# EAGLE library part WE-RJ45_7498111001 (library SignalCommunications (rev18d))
Order Code 7498111001 Design SMD xBase-T 10/100/1000 Base-T Ports 1x1 Application Standard Tab Position UP LED (Left-Right) NONE EMI Fingers Yes Details see: http://katalog.we-online.de/en/pbs/WE-LAN_RJ45/7498111001? Updated by Yingchun Shan 2016-08-23 2014 (C) Würth Elektronik
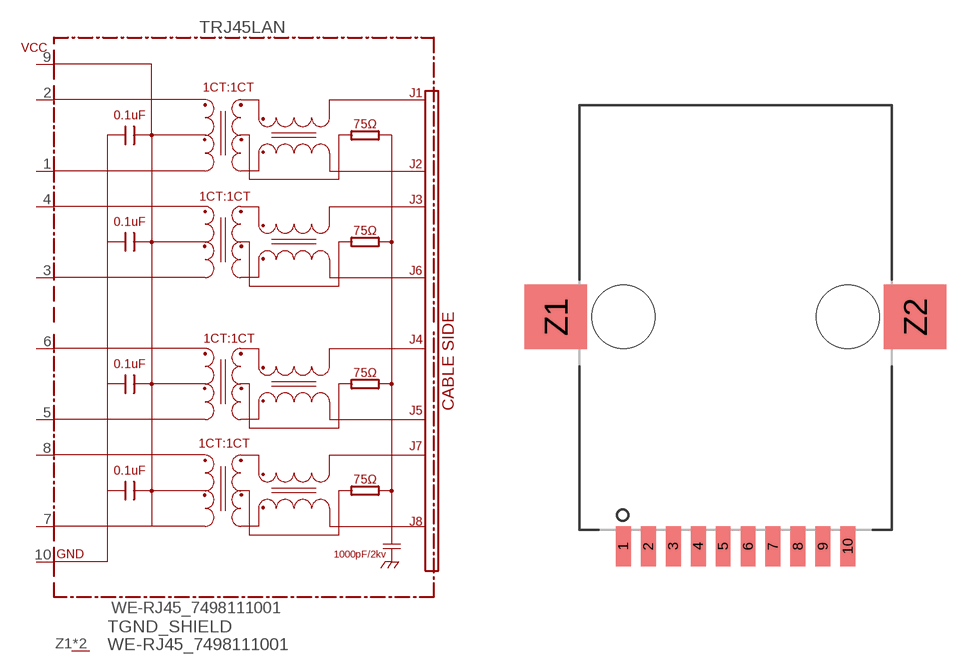
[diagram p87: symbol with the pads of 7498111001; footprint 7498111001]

Designator prefix T; gates RJ45LAN=7498111001 GND_SHIELD=GNDPIN

## WE-RJ45_7498111001 (COMPANY-URL: http://www.we-online.de; CREATED-BY: Christin Zierenner; CREATED-DATE: AUG 2012; DATASHEET-URL: http://katalog.we-online.de/kataloge/eisos/media/pdf/7498111001.pdf; MANUFACTURER: Würth Elektronik eiSos GmbH)  [7498111001]
1  RJ45LAN:1
2  RJ45LAN:2
3  RJ45LAN:3
4  RJ45LAN:4
5  RJ45LAN:5
6  RJ45LAN:6
7  RJ45LAN:7
8  RJ45LAN:8
9  RJ45LAN:VCC
10  RJ45LAN:GND
Z1  GND_SHIELD:GND  pwr
Z2  GND_SHIELD:GND  pwr

## Footprint 7498111001 (pad centres in mm)
MAX HEIGHT=13.55mm PORTS----1X1 LED -NO
smd 0.76 x 2.03: 1 -5.715,-11.68; 2 -4.445,-11.68; 3 -3.175,-11.68; 4 -1.905,-11.68; 5 -0.635,-11.68; 6 0.635,-11.68; 7 1.905,-11.68; 8 3.175,-11.68; 9 4.445,-11.68; 10 5.715,-11.68
smd 3.18 x 3.3: Z1 -9.145,0; Z2 9.145,0
hole 3.22 at 5.715,0
hole 3.22 at -5.715,0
